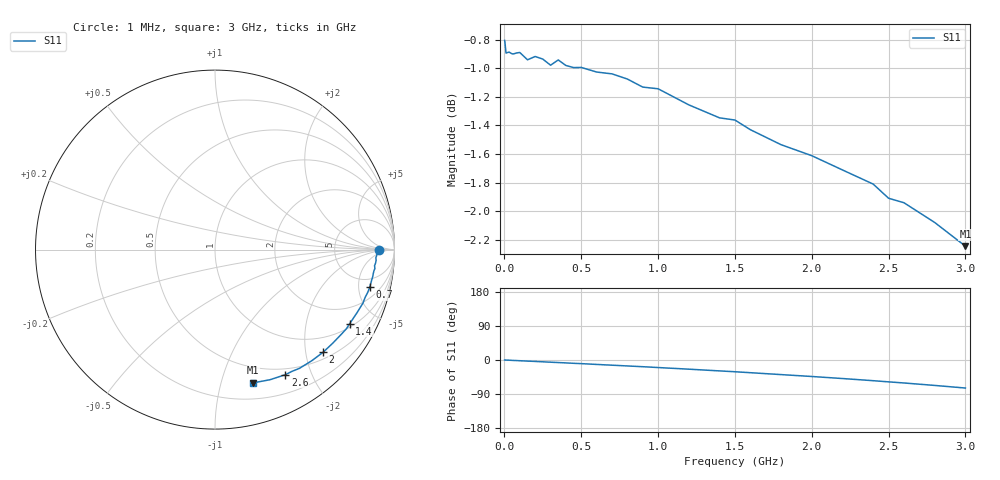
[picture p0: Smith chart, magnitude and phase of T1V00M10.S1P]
! SIEMENS Small Signal Semiconductors
! BAT68-04
! Si Schottky Diode (2 diodes in series, pin 3 open) in SOT23
! IF = 0.1 mA
! S-Parameters:  August  1994
# GHz  S  MA  R  50
!  f  S11
! GHz  MAG  ANG
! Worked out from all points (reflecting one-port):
!   33 points, 1 MHz to 3 GHz, reference 50 ohm
!   lowest |S11| = -2.2 dB at 3 GHz (marker M1), VSWR 7.78, Z = 17.2 - j63.4 ohm
!   phase of S11 starts at 0 deg and turns -74 deg over the sweep
!   S11 on the Smith chart (normalised r, x): 1 MHz: 22, +0; 700 MHz: 3.37, -6.65; 1.4 GHz: 1.15, -3.55; 2 GHz: 0.64, -2.36; 2.6 GHz: 0.42, -1.63; 3 GHz: 0.34, -1.27
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0.001  0.9114 0.0
0.01  0.9022 -0.2
0.03  0.9029 -0.5
0.05  0.9016 -1.0
0.1  0.9026 -1.9
0.15  0.8973 -2.9
0.2  0.8997 -3.8
0.25  0.8978 -4.8
0.3  0.8934 -5.8
0.35  0.8972 -6.7
0.4  0.8932 -7.7
0.5  0.8918 -9.6
0.7  0.8872 -13.7
0.8  0.8835 -15.7
0.9  0.8778 -17.7
1  0.8766 -19.9
1.2  0.8653 -24.2
1.4  0.8563 -28.8
1.5  0.8548 -31.0
1.6  0.8482 -33.5
1.8  0.838 -38.5
2  0.8306 -43.5
2.2  0.8211 -48.9
2.4  0.8118 -54.6
2.5  0.8026 -57.7
2.6  0.7997 -60.6
2.8  0.7871 -67.1
3  0.7722 -74.0
